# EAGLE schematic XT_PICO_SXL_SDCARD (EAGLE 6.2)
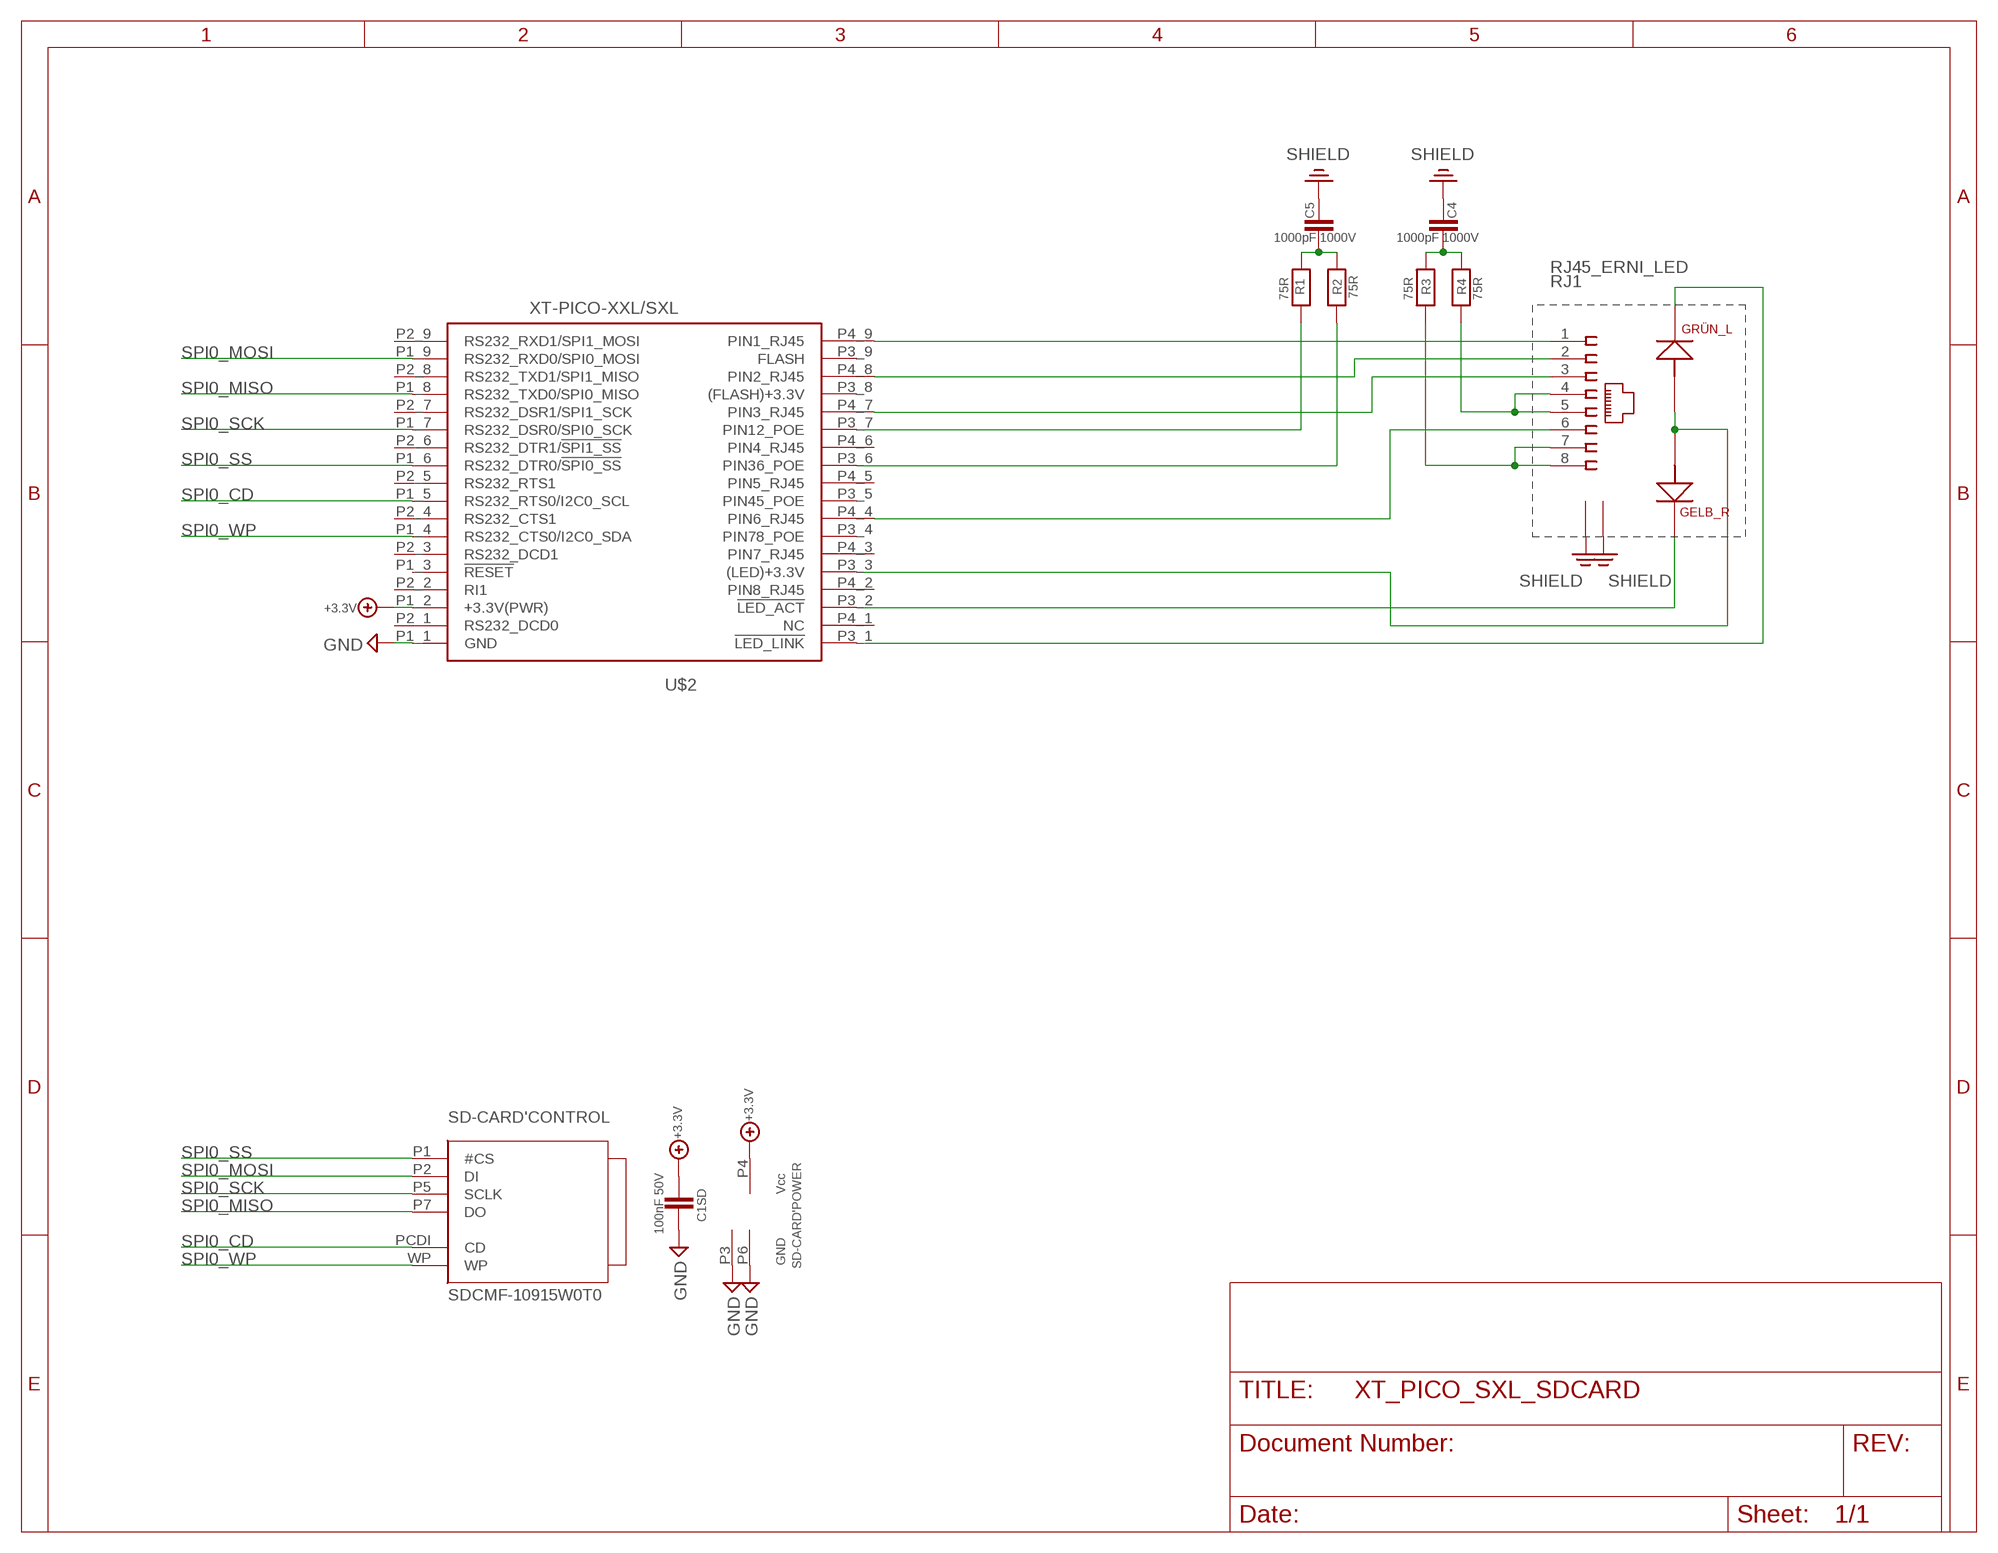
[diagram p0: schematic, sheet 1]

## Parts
C1SD  100nF 50V  CHIP-C-0603  [SMD-0603]
C4  1000pF 1000V  CHIP-C-1210  [SMD-1210]
C5  1000pF 1000V  CHIP-C-1210  [SMD-1210]
R1  75R  CHIP-R-0603  [SMD-0603]
R2  75R  CHIP-R-0603  [SMD-0603]
R3  75R  CHIP-R-0603  [SMD-0603]
R4  75R  CHIP-R-0603  [SMD-0603]
RJ1  RJ45_ERNI_LED  [ORCAD_X_ERNI_RJ45_LED]
SD-CARD  SDCMF-10915W0T0  SDCMF-109XXW010SDCMF-10915W0T1_SO  [SDCMF-10915W0T1]
U$2  XT-PICO-XXL/SXL  [XT-PICO-XXL/SXL]

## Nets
+3.3V: C1SD.2 SD-CARD.P4('POWER:VCC) U$2.P1_2(+3.3V(PWR))
GND: C1SD.1 SD-CARD.P3('POWER:GND) SD-CARD.P6('POWER:GND) U$2.P1_1(GND)
N$1: RJ1.1 U$2.P4_9(PIN1_RJ45)
N$2: RJ1.3 U$2.P4_7(PIN3_RJ45)
N$4: R1.2 U$2.P3_7(PIN12_POE)
N$6: R2.2 U$2.P3_6(PIN36_POE)
N$7: R4.2 RJ1.4 RJ1.5
N$8: RJ1.2 U$2.P4_8(PIN2_RJ45)
N$10: R3.2 RJ1.7 RJ1.8
N$12: RJ1.6 U$2.P4_4(PIN6_RJ45)
N$15: RJ1.A1 RJ1.A2 U$2.P3_3((LED)+3.3V)
N$16: RJ1.K1 U$2.P3_2(!LED_ACT)
N$17: RJ1.K2 U$2.P3_1(!LED_LINK)
N$19: C4.2 R3.1 R4.1
N$20: C5.1 R1.1 R2.1
PE: RJ1.9 RJ1.10 ; supply symbol labelled SHIELD
SHIELD: C4.1 C5.2
SPI0_CD: SD-CARD.PCDI('CONTROL:CD) U$2.P1_5(RS232_RTS0/I2C0_SCL)
SPI0_MISO: SD-CARD.P7('CONTROL:DO) U$2.P1_8(RS232_TXD0/SPI0_MISO)
SPI0_MOSI: SD-CARD.P2('CONTROL:DI) U$2.P1_9(RS232_RXD0/SPI0_MOSI)
SPI0_SCK: SD-CARD.P5('CONTROL:SCLK) U$2.P1_7(RS232_DSR0/SPI0_SCK)
SPI0_SS: SD-CARD.P1('CONTROL:#CS) U$2.P1_6(RS232_DTR0/!SPI0_SS!)
SPI0_WP: SD-CARD.WP('CONTROL:WP) U$2.P1_4(RS232_CTS0/I2C0_SDA)
Unconnected: U$2.P1_3(!RESET) U$2.P2_1(RS232_DCD0) U$2.P2_2(RI1) U$2.P2_3(RS232_DCD1) U$2.P2_4(RS232_CTS1) U$2.P2_5(RS232_RTS1) U$2.P2_6(RS232_DTR1/!SPI1_SS!) U$2.P2_7(RS232_DSR1/SPI1_SCK) U$2.P2_8(RS232_TXD1/SPI1_MISO) U$2.P2_9(RS232_RXD1/SPI1_MOSI) U$2.P3_4(PIN78_POE) U$2.P3_5(PIN45_POE) U$2.P3_8((FLASH)+3.3V) U$2.P3_9(FLASH) U$2.P4_1(NC) U$2.P4_2(PIN8_RJ45) U$2.P4_3(PIN7_RJ45) U$2.P4_5(PIN5_RJ45) U$2.P4_6(PIN4_RJ45)

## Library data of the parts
C1SD = mea-lib:CHIP-C-?: Chip capacitance
C4 C5 = XTMACRO:CHIP-C-?: Chip capacitance
R1-R4 = XTMACRO:CHIP-R-?: Chip resistors
RJ1 = XTMACRO:RJ45_ERNI_LED
SD-CARD = sdcards:SDCMF-109XXW010: KingFont SD-CARD SDCMF-109XXW010 SPI -MODE
U$2 = ak-devices:XT-PICO-XXL/SXL: AK-NORD XT-PICO-XXL/SXL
